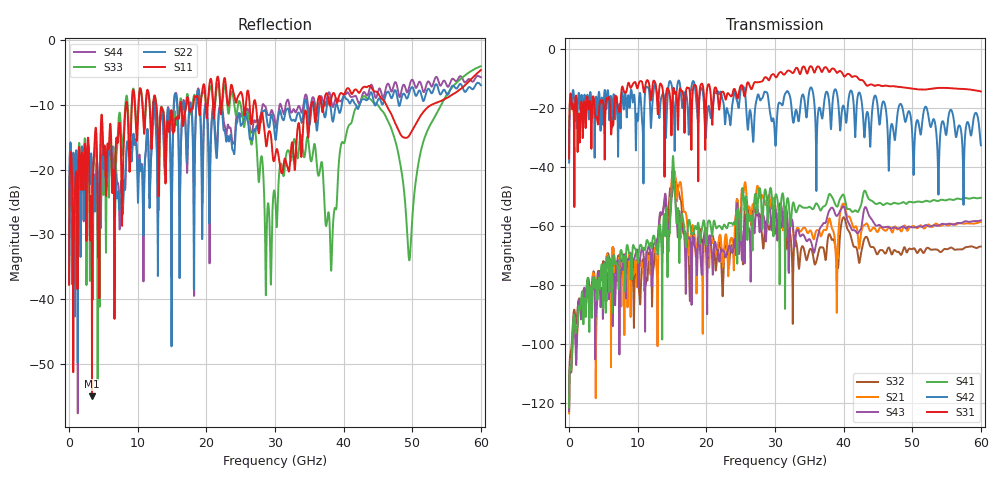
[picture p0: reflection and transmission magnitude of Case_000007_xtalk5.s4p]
! Info: Touchstone file created by circ.  Input file=CasetestDOE_NRZ_template_000007.circ
# Hz S RI R 50
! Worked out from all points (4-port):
!   6000 points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, 10 MHz to 60 GHz, reference 50 ohm
!   strongest paths, dB at 10 MHz, 15.01 GHz, 30.01 GHz, 45.01 GHz, 60 GHz:
!     S31: -37.1, -20.1, -9.2, -12.2, -14.4
!     S42: -38.5, -13.1, -30.5, -20.6, -32.6
!     S41: -121.4, -43.1, -50.5, -52.3, -50.4
!     S43: -122.7, -45.9, -53.0, -59.7, -58.1
!     S21: -123.4, -43.0, -52.3, -61.9, -58.6
!     S32: -120.7, -49.0, -61.8, -69.3, -66.9
!   lowest |S11| = -55.0 dB at 3.34 GHz (marker M1), VSWR 1.00, Z = 50.1 + j0.149 ohm
!   |S11| at or under -10 dB: start of sweep to 8.28 GHz; 27.21 GHz to 35.28 GHz (8.066 GHz wide, 25.8 % of centre); 46.21 GHz to 52.83 GHz (6.613 GHz wide, 13.4 % of centre)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
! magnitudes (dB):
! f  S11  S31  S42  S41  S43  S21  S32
! 10 MHz  -37.8  -37.1  -38.5  -121.4  -122.7  -123.4  -120.7
! 3.34 GHz  -55.0  -21.7  -23.2  -88.5  -82.4  -83.1  -79.3
! 12.75 GHz  -10.5  -14.7  -14.5  -67.4  -65.3  -74.0  -67.8
! 15.24 GHz  -14.0  -13.1  -19.7  -39.4  -44.9  -43.1  -46.2
! 17.62 GHz  -11.1  -15.3  -18.0  -58.9  -64.5  -73.1  -85.0
! 49.57 GHz  -14.7  -13.3  -21.1  -51.8  -60.2  -60.6  -67.6
! 60 GHz  -4.6  -14.4  -32.6  -50.4  -58.1  -58.6  -66.9
